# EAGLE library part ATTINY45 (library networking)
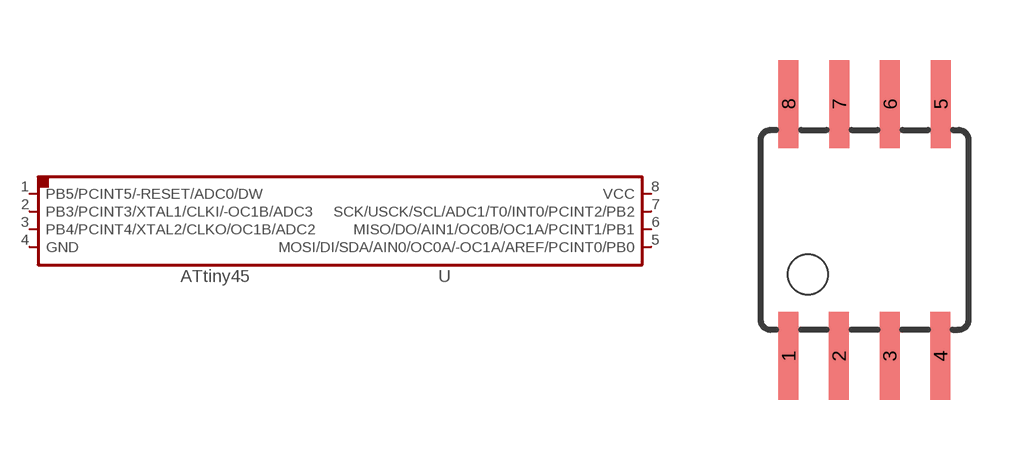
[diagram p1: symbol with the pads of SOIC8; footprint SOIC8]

Designator prefix -

## ATTINY45SI  [SOIC8]
1  PB5/PCINT5/-RESET/ADC0/DW
2  PB3/PCINT3/XTAL1/CLKI/-OC1B/ADC3
3  PB4/PCINT4/XTAL2/CLKO/OC1B/ADC2
4  GND
5  MOSI/DI/SDA/AIN0/OC0A/-OC1A/AREF/PCINT0/PB0
6  MISO/DO/AIN1/OC0B/OC1A/PCINT1/PB1
7  SCK/USCK/SCL/ADC1/T0/INT0/PCINT2/PB2
8  VCC

## Footprint SOIC8 (pad centres in mm)
Wide Plastic Gull Wing Small Outline Package
smd 0.5 x 2.2: 1 -1.905,-3.154; 2 -0.645,-3.154; 3 0.625,-3.154; 4 1.895,-3.154; 5 1.905,3.154; 6 0.635,3.154; 7 -0.635,3.154; 8 -1.905,3.154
